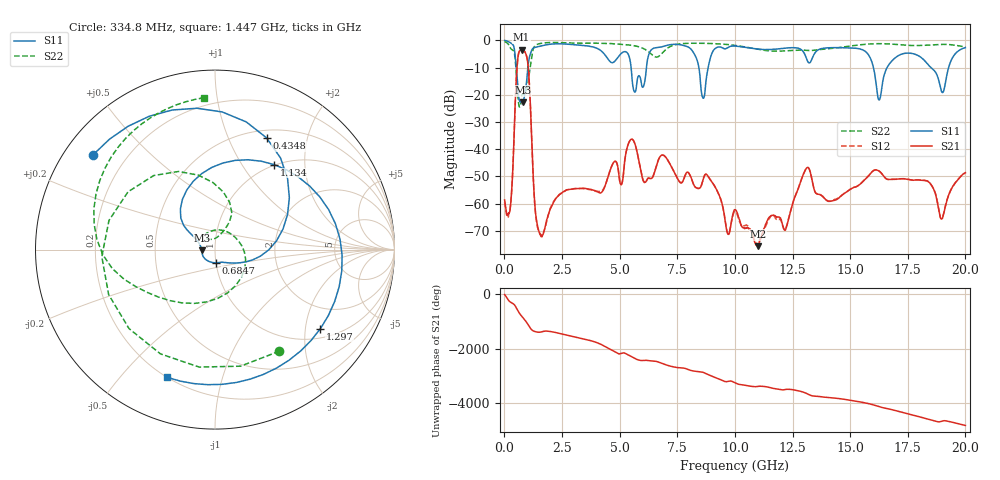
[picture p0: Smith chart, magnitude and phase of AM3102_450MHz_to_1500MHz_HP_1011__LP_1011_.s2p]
!Agilent Technologies,E8364B,MY43040894,A.07.50.67
!Agilent E8364B: A.07.50.67
!Date: Thursday, January 11, 2018 06:25:49
!Correction: S11(Full 2 Port(1,2))
!S21(Full 2 Port(1,2))
!S12(Full 2 Port(1,2))
!S22(Full 2 Port(1,2))
!S2P File: Measurements: S11, S21, S12, S22:
# Hz S  dB  R 50
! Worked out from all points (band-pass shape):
!   1601 points, 10 MHz to 20 GHz, reference 50 ohm
!   highest |S21| = -3.44 dB at 747.1 MHz (marker M1); lowest = -75.6 dB at 11 GHz (marker M2)
!   |S21| within 3 dB of the highest: 586.3 MHz to 980.3 MHz (394 MHz wide, 50.3 % of centre)
!   lowest |S11| = -22.7 dB at 797.1 MHz (marker M3), VSWR 1.16, Z = 43.2 - j0.361 ohm
!   |S11| at or under -10 dB: 5.498 GHz to 6.163 GHz (664.9 MHz wide, 11.4 % of centre); 16.01 GHz to 16.6 GHz (593.8 MHz wide, 3.64 % of centre); 18.5 GHz to 19.27 GHz (767.8 MHz wide, 4.06 % of centre)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
!   |S22| runs from -24.5 to -0.5 dB; largest |S21 - S12| = 0.00063
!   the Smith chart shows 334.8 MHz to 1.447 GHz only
!   S11 on the Smith chart (normalised r, x): 334.8 MHz: 0.08, +0.34; 434.8 MHz: 0.59, +1.39; 684.7 MHz: 1.00, -0.15; 1.134 GHz: 0.99, +1.40; 1.297 GHz: 1.27, -2.42; 1.447 GHz: 0.20, -0.68
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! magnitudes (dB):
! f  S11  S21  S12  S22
! 10 MHz  -0.1  -58.6  -59.5  -0.5
! 334.8 MHz  -1.3  -52.7  -52.4  -3.5
! 434.8 MHz  -3.3  -31.4  -31.4  -4.7
! 684.7 MHz  -22.7  -3.6  -3.6  -24.1
! 747.1 MHz  -22.4  -3.4  -3.4  -20.8
! 797.1 MHz  -22.7  -3.5  -3.5  -19.8
! 1.134 GHz  -4.8  -25.1  -25.1  -9.1
! 1.297 GHz  -2.7  -57.4  -57.7  -2.4
! 1.447 GHz  -2.4  -68.5  -68.9  -1.4
! 3.346 GHz  -1.9  -54.4  -54.5  -1.1
! 5.657 GHz  -19.0  -37.9  -37.9  -2.0
! 6.682 GHz  -2.6  -43.9  -44.0  -6.0
! 8.093 GHz  -3.2  -50.2  -50.4  -1.1
! 8.618 GHz  -21.3  -51.2  -51.2  -1.1
! 10.01 GHz  -2.1  -62.2  -62.9  -1.9
! 11 GHz  -3.2  -75.6  -74.7  -3.3
! 13.34 GHz  -6.9  -51.1  -51.1  -3.7
! 15.59 GHz  -3.7  -51.6  -51.5  -1.5
! 16.25 GHz  -21.9  -48.0  -48.0  -1.2
! 16.68 GHz  -9.0  -51.1  -51.1  -1.3
! 18.98 GHz  -18.9  -65.6  -65.6  -1.5
! 20 GHz  -2.7  -48.6  -48.8  -2.4
